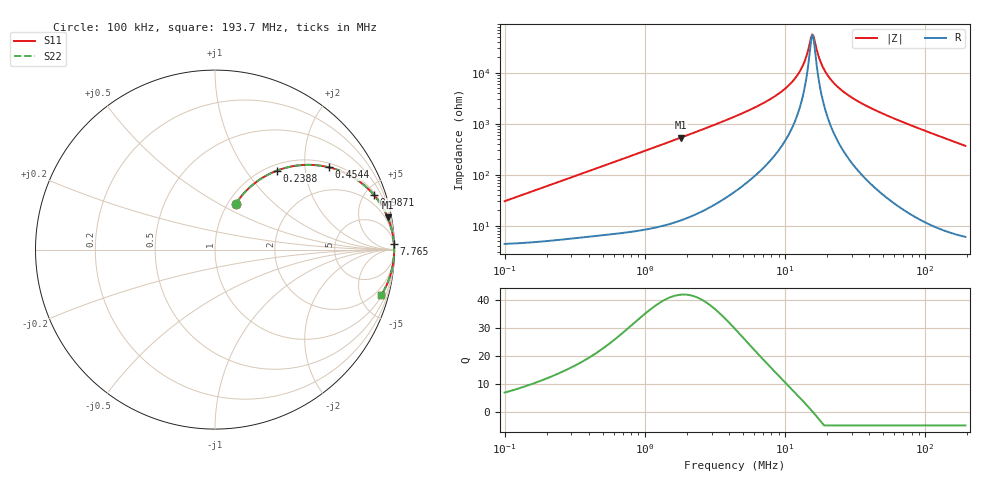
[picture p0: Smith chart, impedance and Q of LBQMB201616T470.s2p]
! LBQMB201616T470  S-PARAMETER MODEL  ( General Type )
! Model Generated by TAIYO YUDEN Corporation (http://www.ty-top.com)
! Version 1.0
! TAIYO YUDEN Control No. 191025NI43SB-FBB
! Copyright(c) 2019 TAIYO YUDEN CO.,LTD. All Rights Reserved.
! Product Description (link to TY-COMPAS)
! https://ds.yuden.co.jp/TYCOMPAS/or/detail?pn=LBQMB201616T470J&u=M
! Products Name : Inductors
! Characteristics :
!  Inductance : 47 uH , SRF(min) : 13 MHz , DC Resistance(max) : 5.33 Ohm , Rated Current : 115 mA
!  Case Size : 2.0 x 1.6 / 0.079 x 0.063 [mm/inch] , Thickness : 1.6 / 0.063 [mm/inch]
!  (Conditions: Temperature = 25 degC , DC Bias Current/Voltage = 0A / 0V)
! External Node Assignments :
!  1  o---GGG---o  2
! GND o---------o GND
! Frequency Range : 0.1MHz  -  193.730505MHz  [ 402 STEP ]
# MHz S RI R 50
! Freq[MHz].  S11 Real  S11 Imag  S21 Real  S21 Imag  S12 Real  S12 Imag  S22 Real  S22 Imag
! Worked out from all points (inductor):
!   401 points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, 100 kHz to 193.7 MHz, reference 50 ohm
!   read as one part in series: L = 47.5 uH near 103.9 kHz
!   highest Q = 42.1 at 1.809 MHz (marker M1), where L = 46.9 uH
!   self-resonance near 15.64 MHz
!   S11 on the Smith chart (normalised r, x): 100 kHz: 1.09, +0.60; 238.8 kHz: 1.10, +1.42; 454.4 kHz: 1.13, +2.67; 987.1 kHz: 1.17, +5.78; 7.765 MHz: 5, +59; 193.7 MHz: 1.12, -7.35
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0.1  0.1145 0.2535  0.8855 -0.2535  0.8855 -0.2535  0.1145 0.2535
0.15453  0.1996 0.352  0.8004 -0.352  0.8004 -0.352  0.1996 0.352
0.238796  0.3456 0.4401  0.6544 -0.4401  0.6544 -0.4401  0.3456 0.4401
0.355309  0.5226 0.4723  0.4774 -0.4723  0.4774 -0.4723  0.5226 0.4723
0.454401  0.6351 0.4584  0.3649 -0.4584  0.3649 -0.4584  0.6351 0.4584
0.987137  0.8863 0.3034  0.1137 -0.3034  0.1137 -0.3034  0.8863 0.3034
1.262442  0.9265 0.2484  0.0735 -0.2484  0.0735 -0.2484  0.9265 0.2484
1.808645  0.9621 0.1794  0.0379 -0.1794  0.0379 -0.1794  0.9621 0.1794
4.401483  0.9925 0.0713  0.00754 -0.0713  0.00754 -0.0713  0.9925 0.0713
7.764953  0.9968 0.0334  0.00317 -0.0334  0.00317 -0.0334  0.9968 0.0334
10.12024  0.9977 0.0199  0.00233 -0.0199  0.00233 -0.0199  0.9977 0.0199
12.22843  0.998 0.0111  0.00198 -0.0111  0.00198 -0.0111  0.998 0.0111
13.69868  0.9982 0.00604  0.00185 -0.00604  0.00185 -0.00604  0.9982 0.00604
15.05805  0.9982 0.00187  0.00178 -0.00187  0.00178 -0.00187  0.9982 0.00187
15.63884  0.9982 0.000212  0.00176 -0.000212  0.00176 -0.000212  0.9982 0.000212
16.24204  0.9983 -0.00145  0.00175 0.00145  0.00175 0.00145  0.9983 -0.00145
17.51913  0.9983 -0.00479  0.00174 0.00479  0.00174 0.00479  0.9983 -0.00479
18.89664  0.9982 -0.00816  0.00176 0.00816  0.00176 0.00816  0.9982 -0.00816
22.83308  0.9981 -0.0168  0.00192 0.0168  0.00192 0.0168  0.9981 -0.0168
32.09878  0.9972 -0.0342  0.00276 0.0342  0.00276 0.0342  0.9972 -0.0342
55.56615  0.9932 -0.0716  0.00683 0.0716  0.00683 0.0716  0.9932 -0.0716
193.7305  0.9276 -0.2512  0.0724 0.2512  0.0724 0.2512  0.9276 -0.2512
